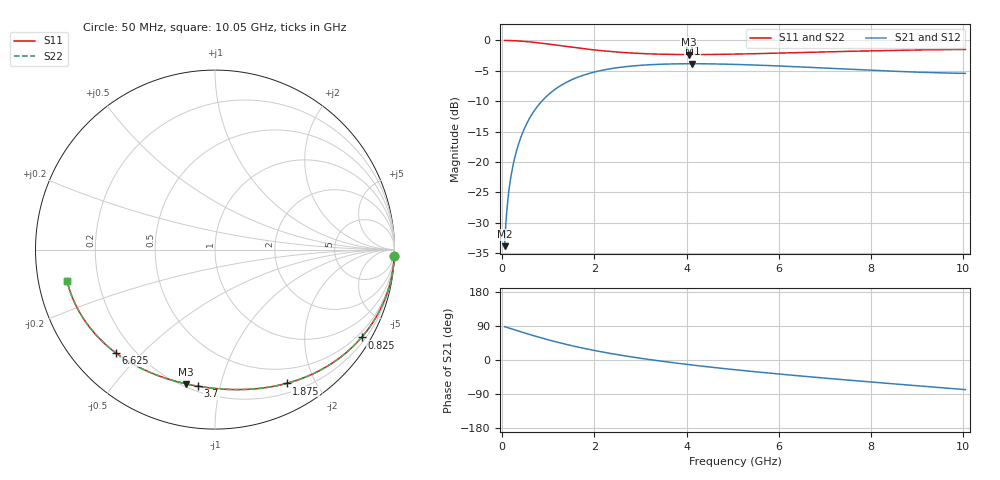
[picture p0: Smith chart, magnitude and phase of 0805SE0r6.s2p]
! AVX Thin Film Operation		Date: August 2001
! Description: Accu-P® Series, Thin Film, SMD, RF Capacitor
! Part Number: 08051J0R6ABT
! 50 MHz  -  10.05 GHz
! Serial Measurements
# mhz S db R 50
!	S11		S21		S12		S22
!	dB	Phase	dB	Phase	dB	Phase	dB	Phase
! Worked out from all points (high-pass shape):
!   401 points, 50 MHz to 10.05 GHz, reference 50 ohm
!   highest |S21| = -3.83 dB at 4.125 GHz (marker M1); lowest = -33.9 dB at 50 MHz (marker M2)
!   |S21| within 3 dB of the highest: 1.406 GHz to end of sweep
!   lowest |S11| = -2.3 dB at 4.05 GHz (marker M3), VSWR 7.52, Z = 10.9 - j39.2 ohm
!   |S11| at or under -10 dB: nowhere
!   |S22| runs from -2.3 to 0.0 dB; largest |S21 - S12| = 0
!   S11 on the Smith chart (normalised r, x): 50 MHz: 0, -59; 825 MHz: 0.34, -3.58; 1.875 GHz: 0.31, -1.63; 3.7 GHz: 0.23, -0.86; 6.625 GHz: 0.13, -0.42; 10.05 GHz: 0.09, -0.10
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50  -0.00 -2.0  -33.88 88.0  -33.88 88.0  -0.00 -2.0
75  -0.00 -2.9  -30.36 87.1  -30.36 87.1  -0.00 -2.9
125  -0.01 -4.9  -25.93 85.1  -25.93 85.1  -0.01 -4.9
175  -0.02 -6.8  -23.03 83.2  -23.03 83.2  -0.02 -6.8
225  -0.04 -8.8  -20.87 81.2  -20.87 81.2  -0.04 -8.8
300  -0.06 -11.7  -18.42 78.3  -18.42 78.3  -0.06 -11.7
400  -0.11 -15.5  -16.00 74.5  -16.00 74.5  -0.11 -15.5
525  -0.19 -20.2  -13.77 69.8  -13.77 69.8  -0.19 -20.2
825  -0.43 -30.9  -10.28 59.1  -10.28 59.1  -0.43 -30.9
1250  -0.85 -44.7  -7.51 45.3  -7.51 45.3  -0.85 -44.7
1725  -1.32 -58.1  -5.81 31.9  -5.81 31.9  -1.32 -58.1
1875  -1.46 -61.9  -5.45 28.1  -5.45 28.1  -1.46 -61.9
2600  -1.97 -77.9  -4.38 12.1  -4.38 12.1  -1.97 -77.9
3400  -2.26 -92.2  -3.93 -2.3  -3.93 -2.3  -2.26 -92.2
3700  -2.30 -97.0  -3.87 -7.0  -3.87 -7.0  -2.30 -97.0
4050  -2.32 -102.2  -3.84 -12.3  -3.84 -12.3  -2.32 -102.2
4125  -2.32 -103.3  -3.83 -13.3  -3.83 -13.3  -2.32 -103.3
5050  -2.25 -115.6  -3.94 -25.7  -3.94 -25.7  -2.25 -115.6
6625  -1.96 -133.8  -4.41 -43.8  -4.41 -43.8  -1.96 -133.8
6725  -1.94 -134.8  -4.45 -44.9  -4.45 -44.9  -1.94 -134.8
8400  -1.65 -151.9  -5.04 -62.0  -5.04 -62.0  -1.65 -151.9
10050  -1.49 -168.0  -5.42 -78.2  -5.42 -78.2  -1.49 -168.0
